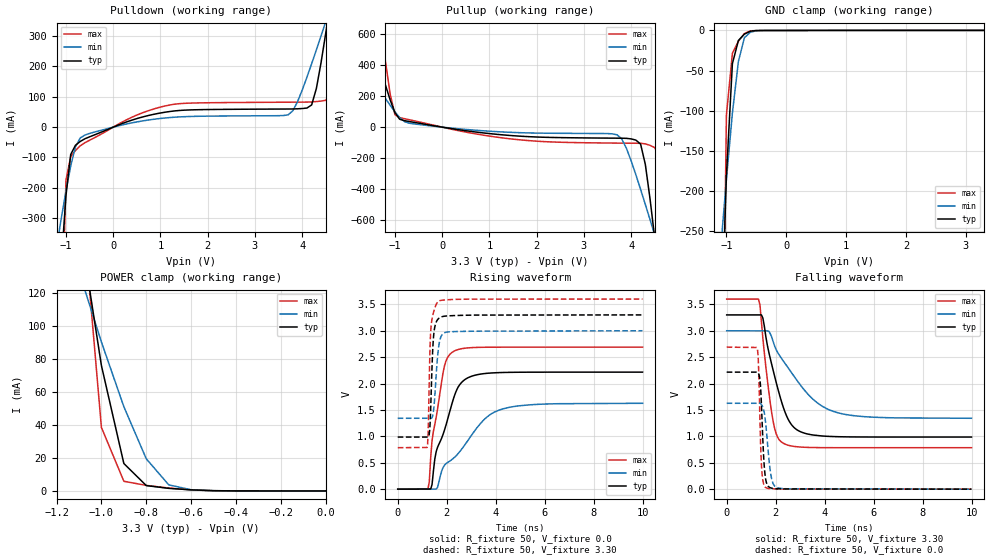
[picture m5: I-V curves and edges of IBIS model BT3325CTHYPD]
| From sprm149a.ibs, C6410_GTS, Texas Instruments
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[Model]   BT3325CTHYPD
Model_type   I/O
Vinh = 2.00
Vinl = 0.80
Enable   Active-Low
Polarity   Non-Inverting
| signals   A, GZ, Y
Vmeas = 1.5
|   typ   min   max
C_comp   1.5797p   1.5046p   1.7659p
|   typ   min   max
[Temperature Range]   25   -40   125
|   typ   min   max
[Voltage Range]   3.30V   3.00V   3.60V
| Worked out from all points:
|   slope of the pulldown table from 0 to 0.495 V, typ, clamps not added: 17.7 ohm
|   slope of the pullup table from 0 to 0.495 V, typ, clamps not added: 21.6 ohm
|   GND clamp passes 1 mA (typ) near -0.60 V on its own axis
|   POWER clamp passes 1 mA (typ) near -0.64 V on its own axis
|   rising waveform, R_fixture 50, V_fixture 0.0: 20-80 % time 838ps typ, 1.71ns min, 494ps max; typ from 0 V to 2.22 V
|   falling waveform, R_fixture 50, V_fixture 3.30: 20-80 % time 773ps typ, 1.6ns min, 430ps max; typ from 3.3 V to 0.987 V
|   rising waveform, R_fixture 50, V_fixture 3.30: 20-80 % time 114ps typ, 164ps min, 98.9ps max; typ from 0.987 V to 3.3 V
|   falling waveform, R_fixture 50, V_fixture 0.0: 20-80 % time 131ps typ, 208ps min, 99.4ps max; typ from 2.22 V to 0 V
[Pulldown]
|   Voltage   I(typ)   I(min)   I(max)
-3.3V     -6.793A    -2.574A    -22.74A
-1.1V     -450.2mA   -301.1mA   -721mA
-900mV    -90.07mA   -128.3mA   -97.37mA
-600mV    -38.44mA   -26.14mA   -51.28mA
1.2V      51.55mA    31.56mA    73.11mA
3.7V      59.71mA    40.51mA    82.18mA
4.2V      73.19mA    209.1mA    83.11mA
4.5V      311.5mA    348.4mA    88.34mA
4.6V      414.6mA    395.8mA    114.7mA
4.7V      520.6mA    443.6mA    265.1mA
4.8V      628.2mA    491.6mA    481.3mA
6.6V      2.638A     1.372A     5.219A
[GND_clamp]
|   Voltage   I(typ)   I(min)   I(max)
-3.3V     -6.736A    -2.536A    -22.69A
-1.1V     -409mA     -276.3mA   -663.3mA
-1V       -181.3mA   -185.6mA   -105.8mA
-900mV    -41.31mA   -103mA     -28.49mA
-800mV    -12.56mA   -38.78mA   -13.44mA
-700mV    -4.536mA   -9.107mA   -3.884mA
-600mV    -909.4uA   -2.154mA   -504.7uA
-400mV    -40.5uA    -67.44uA   -56.49uA
3.3V      100.9uA    54.24uA    177.6uA
[Pullup]
|   Voltage   I(typ)   I(min)   I(max)
-3.3V     2.592A     1.197A     5.962A
-2.2V     1.358A     659mA      3.009A
-1.6V     694.5mA    370.4mA    1.423A
-1.3V     373.4mA    230mA      660.8mA
-1V       93.76mA    98.94mA    81.03mA
-800mV    41.96mA    36.18mA    54.78mA
3.7V      -71.34mA   -49.46mA   -103.2mA
4.1V      -83.89mA   -308.4mA   -104.2mA
4.5V      -721.3mA   -699.1mA   -132.7mA
4.6V      -990.6mA   -800.1mA   -203.9mA
4.7V      -1.267A    -901.8mA   -745.3mA
6.6V      -6.788A    -2.882A    -19.69A
[POWER_clamp]
|   Voltage   I(typ)   I(min)   I(max)
-3.3V     2.586A     1.19A      5.96A
-1.1V     163.9mA    133.1mA    196.9mA
-1V       76.05mA    90.34mA    38.49mA
-900mV    16.63mA    51.08mA    5.85mA
-800mV    3.238mA    19.47mA    3.36mA
-700mV    1.562mA    3.689mA    1.736mA
-600mV    653.8uA    701.7uA    607.7uA
-500mV    154.7uA    155.6uA    89.49uA
0V        1pA        1pA        1pA
[Ramp]
|   I(typ)   I(min)   I(max)
dV/dt_r   1.330/0.840n   0.976/1.712n   1.613/0.493n
dV/dt_f   1.388/0.774n   0.995/1.601n   1.689/0.431n
[Rising Waveform]
R_fixture = 50
V_fixture = 0.0
|  pu_on
|  TIME   V(typ)   V(min)   V(max)
0s        2nV        11nV       1nV
1.234ns   2.498mV    1.679mV    1.38nV
1.29ns    2.498mV    1.841mV    140mV
1.402ns   88.19mV    1.841mV    920.7mV
1.57ns    710.4mV    1.841mV    1.362V
1.851ns   1.037V     408.5mV    2.203V
2.3ns     1.747V     594.6mV    2.613V
2.862ns   2.108V     919.3mV    2.675V
4.321ns   2.21V      1.524V     2.689V
10ns      2.216V     1.626V     2.689V
[Falling Waveform]
R_fixture = 50
V_fixture = 3.30
V_fixture_min = 3.00
V_fixture_max = 3.60
|  pd_on
|  TIME   V(typ)   V(min)   V(max)
0s        3.3V       3V         3.6V
1.298ns   3.3V       2.998V     3.6V
1.358ns   3.3V       2.998V     3.492V
1.479ns   3.239V     2.998V     2.854V
1.9ns     2.247V     2.79V      1.277V
2.081ns   1.917V     2.59V      983.3mV
2.322ns   1.538V     2.422V     868.4mV
2.924ns   1.109V     2.026V     800.8mV
4.49ns    994.4mV    1.454V     785.5mV
10ns      986.8mV    1.342V     785.2mV
[Rising Waveform]
R_fixture = 50
V_fixture = 3.30
V_fixture_min = 3.00
V_fixture_max = 3.60
|  pd_off
|  TIME   V(typ)   V(min)   V(max)
0s        986.8mV    1.342V     785.2mV
1.2ns     986.8mV    1.343V     790.5mV
1.241ns   986.8mV    1.343V     1.058V
1.303ns   1.107V     1.343V     2.402V
1.365ns   1.797V     1.343V     3.097V
1.427ns   2.614V     1.387V     3.283V
1.468ns   2.916V     1.514V     3.358V
1.674ns   3.233V     2.702V     3.56V
2.044ns   3.281V     2.978V     3.587V
10ns      3.3V       3V         3.6V
[Falling Waveform]
R_fixture = 50
V_fixture = 0.0
|  pu_off
|  TIME   V(typ)   V(min)   V(max)
0s        2.216V     1.626V     2.689V
1.252ns   2.216V     1.626V     2.654V
1.304ns   2.185V     1.626V     2.286V
1.356ns   2.083V     1.626V     1.352V
1.434ns   1.431V     1.592V     354.6mV
1.525ns   495.4mV    1.473V     77.47mV
1.603ns   162.2mV    1.198V     28.81mV
1.812ns   22.27mV    253.9mV    8.346mV
2.072ns   7.517mV    27.39mV    4.656mV
10ns      473.5nV    5.39uV     259.4nV
